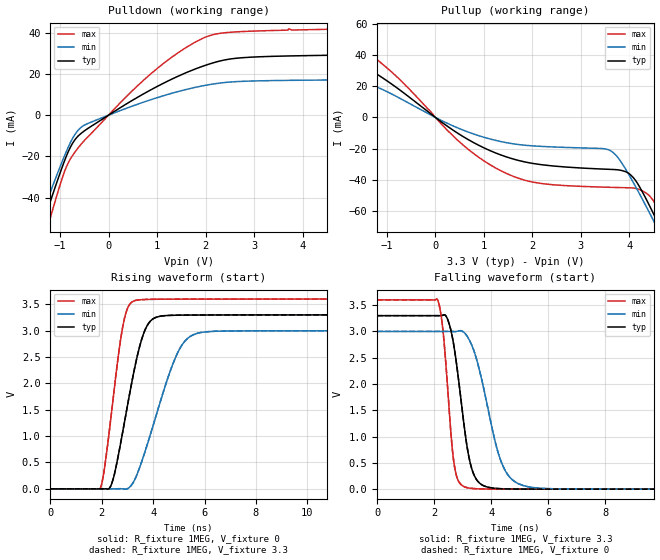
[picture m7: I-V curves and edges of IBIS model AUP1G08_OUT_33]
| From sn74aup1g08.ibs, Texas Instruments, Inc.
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[Model]   AUP1G08_OUT_33
Model_type  Output
Vref =   0
Rref =   1E6
Cref =   30p
Vmeas =   1.65
| variable   typ   min   max
C_comp   2.86pF   1.97pF   4.18pF
| C_pullup   3.23pF   1.97pF   4.18pF
| C_pulldown   2.49pF   2.28pF   3.06pF
[Temperature Range]   40   100   -40
| Ambient temperature   25   85   -40
[Voltage range]   3.3   3   3.6
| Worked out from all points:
|   slope of the pulldown table from 0 to 0.495 V, typ, clamps not added: 68.4 ohm
|   slope of the pullup table from 0 to 0.495 V, typ, clamps not added: 45.8 ohm
|   rising waveform, R_fixture 1MEG, V_fixture 0: 20-80 % time 788ps typ, 1.18ns min, 552ps max; typ from 0 V to 3.3 V
|   falling waveform, R_fixture 1MEG, V_fixture 3.3: 20-80 % time 485ps typ, 775ps min, 311ps max; typ from 3.3 V to 0 V
|   rising waveform, R_fixture 1MEG, V_fixture 3.3: 20-80 % time 787ps typ, 1.18ns min, 552ps max; typ from 0 V to 3.3 V
|   falling waveform, R_fixture 1MEG, V_fixture 0: 20-80 % time 485ps typ, 775ps min, 311ps max; typ from 3.3 V to 0 V
[Pulldown]
| AUP1G08_OUT_33
|   Voltage   I(typ)   I(min)   I(max)
-3.6V     -218.8mA   -196.4mA   -248.7mA
-1.515V   -64.4mA    -57.35mA   -75.85mA
-1.39V    -55.38mA   -49.33mA   -65.43mA
-1.275V   -47.16mA   -42.02mA   -55.91mA
-870mV    -19.94mA   -17.64mA   -25.18mA
-720mV    -12.86mA   -10.38mA   -18.82mA
-545mV    -8.444mA   -5.51mA    -13.51mA
940mV     13.13mA    8.018mA    21.36mA
1.5V      19.56mA    11.86mA    31.27mA
2.045V    24.53mA    14.67mA    38.2mA
3.1V      28.27mA    16.63mA    40.81mA
7.2V      29.73mA    17.36mA    42.67mA
[Pullup]
| AUP1G08_OUT_33
|   Voltage   I(typ)   I(min)   I(max)
-3.6V     42.87mA    27.21mA    57.96mA
-2.465V   31.52mA    19.46mA    45.92mA
-1.53V    32.86mA    22.06mA    44.96mA
-755mV    18.1mA     12.64mA    24.89mA
555mV     -11.98mA   -7.942mA   -17.3mA
1.65V     -27.07mA   -17.13mA   -38.31mA
3.61V     -33.32mA   -21.39mA   -44.82mA
4.08V     -38.64mA   -41.79mA   -45.28mA
4.375V    -54.27mA   -58.93mA   -49.24mA
4.565V    -66.26mA   -70.41mA   -57.33mA
4.775V    -80.05mA   -83.34mA   -71.38mA
7.2V      -250.9mA   -241mA     -257.1mA
[Ramp]
| AUP1G08_OUT_33
| variable   typ   min   max
dV/dt_r   1.98/7.89E-10   1.80/1.18E-09   2.16/5.53E-10
dV/dt_f   1.99/4.92E-10   1.81/7.81E-10   2.17/3.16E-10
R_load = 1MEG
[Rising Waveform]
| AUP1G08_OUT_33
R_fixture =   1MEG
C_fixture =   0
L_fixture =   0
V_fixture =   0
V_fixture_min = 0
V_fixture_max = 0
|   Time   V(typ)   V(min)   V(max)
0s        30.39nV    108nV      2.402nV
1.95ns    -47.02uV   1.246uV    16.92mV
2.38ns    85.47mV    -106.5uV   1.437V
2.82ns    1.085V     -527.3uV   3.075V
3.325ns   2.389V     214.9mV    3.575V
3.645ns   2.964V     645.4mV    3.591V
3.975ns   3.216V     1.159V     3.595V
4.965ns   3.294V     2.59V      3.598V
5.795ns   3.297V     2.96V      3.599V
29.99ns   3.3V       3V         3.6V
[Falling Waveform]
| AUP1G08_OUT_33
R_fixture =   1MEG
C_fixture =   0
L_fixture =   0
V_fixture =   3.3
V_fixture_min = 3
V_fixture_max = 3.6
|   Time   V(typ)   V(min)   V(max)
0s        3.3V       3V         3.6V
2.125ns   3.3V       3V         3.595V
2.32ns    3.312V     3V         2.953V
2.505ns   3.179V     3V         1.678V
2.71ns    2.661V     2.997V     439.8mV
3.18ns    723.6mV    2.888V     25.61mV
3.53ns    149.4mV    2.386V     6.907mV
4.37ns    8.037mV    493.6mV    632.6uV
5.285ns   942.5uV    46.5mV     194.2uV
29.99ns   216.8uV    320.7uV    141.5uV
[Rising Waveform]
| AUP1G08_OUT_33
R_fixture =   1MEG
C_fixture =   0
L_fixture =   0
V_fixture =   3.3
V_fixture_min = 3
V_fixture_max = 3.6
|   Time   V(typ)   V(min)   V(max)
0s        216.3uV    319.9uV    141.3uV
1.95ns    169.3uV    321uV      17.07mV
2.38ns    85.73mV    213.3uV    1.437V
2.82ns    1.086V     -207.1uV   3.076V
3.325ns   2.39V      215.5mV    3.576V
3.645ns   2.965V     646.4mV    3.591V
3.975ns   3.217V     1.161V     3.595V
4.965ns   3.294V     2.591V     3.599V
5.795ns   3.297V     2.96V      3.599V
29.99ns   3.3V       3V         3.6V
[Falling Waveform]
| AUP1G08_OUT_33
R_fixture =   1MEG
C_fixture =   0
L_fixture =   0
V_fixture =   0
V_fixture_min = 0
V_fixture_max = 0
|   Time   V(typ)   V(min)   V(max)
0s        3.3V       3V         3.6V
2.125ns   3.3V       3V         3.595V
2.32ns    3.312V     3V         2.953V
2.505ns   3.179V     3V         1.677V
2.71ns    2.661V     2.997V     439.4mV
3.18ns    722.9mV    2.888V     25.45mV
3.53ns    149mV      2.385V     6.761mV
4.37ns    7.807mV    492.7mV    490.6uV
5.285ns   723.5uV    46.05mV    52.81uV
29.99ns   519.5nV    926.6nV    207.9nV
